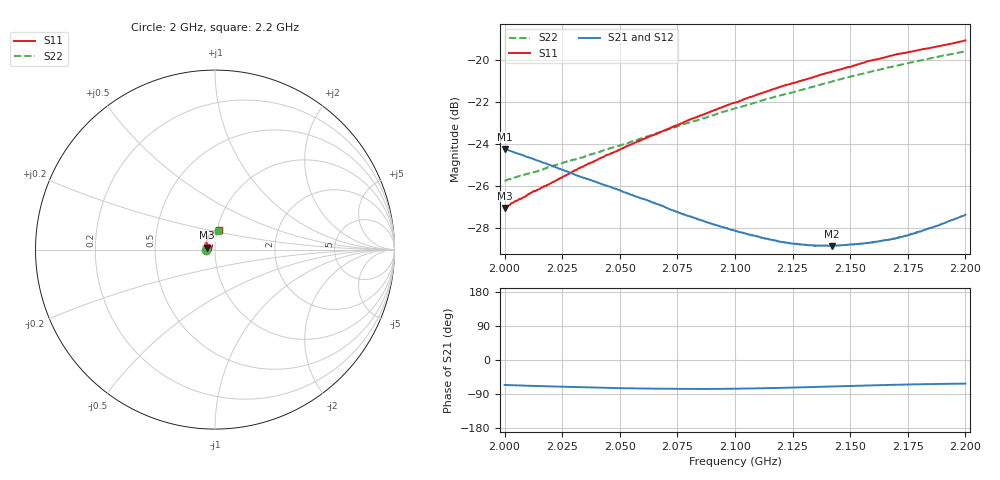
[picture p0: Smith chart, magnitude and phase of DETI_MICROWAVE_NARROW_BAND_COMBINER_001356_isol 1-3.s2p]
! 12/28/2020 4:17:23 PM
! \\DETI-AD\SERVEUR COMMUN\0\01 - PRODUIT\0 01 356 - COMBINEUR 4 VOIES BANDE S 800 WATTS\81 -PROCES VERBAL DE CONTROLE\MESURES\07 - S2P\ISOL 1-3.S2P
! CHANNEL.1
! TR.MEASUREMENT
! CORRECTED.DATA
# GHZ S RI R 50.0
! FREQ.GHZ  S11RE  S11IM  S21RE  S21IM  S12RE  S12IM  S22RE  S22IM
!; PortSelection: Port_12
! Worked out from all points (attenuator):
!   1000 points, 2 GHz to 2.2 GHz, reference 50 ohm
!   highest |S21| = -24.23 dB at 2 GHz (marker M1); lowest = -28.8 dB at 2.142 GHz (marker M2)
!   lowest |S11| = -27.0 dB at 2 GHz (marker M3), VSWR 1.09, Z = 45.9 + j1.04 ohm
!   |S11| at or under -10 dB: start of sweep to end of sweep
!   |S22| runs from -25.7 to -19.6 dB; largest |S21 - S12| = 0.00038
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2  -0.043 0.0113  0.0252 -0.056  0.0252 -0.0562  -0.0517 0.000494
2.011812  -0.0451 0.0178  0.0216 -0.0542  0.0218 -0.0543  -0.0535 0.00736
2.018619  -0.0456 0.0217  0.0199 -0.0529  0.0199 -0.0531  -0.0542 0.0117
2.033433  -0.0467 0.0302  0.0163 -0.0501  0.0163 -0.0504  -0.0548 0.0205
2.044244  -0.0468 0.0366  0.0143 -0.0482  0.0143 -0.0483  -0.0547 0.0275
2.052853  -0.0463 0.0416  0.0129 -0.0466  0.0129 -0.0467  -0.0541 0.0329
2.066667  -0.0448 0.0499  0.0113 -0.044  0.0113 -0.044  -0.0525 0.0418
2.074675  -0.0434 0.0547  0.0105 -0.0423  0.0105 -0.0424  -0.0511 0.0469
2.079279  -0.0426 0.0576  0.0101 -0.0415  0.0102 -0.0417  -0.0501 0.0499
2.1001  -0.037 0.0698  0.0097 -0.0381  0.00975 -0.0383  -0.0441 0.0627
2.116116  -0.0313 0.079  0.0103 -0.0359  0.0102 -0.0361  -0.0376 0.072
2.120521  -0.0295 0.0813  0.0105 -0.0354  0.0104 -0.0356  -0.0357 0.0743
2.128929  -0.0256 0.0853  0.0111 -0.0347  0.0111 -0.0349  -0.0313 0.0787
2.133534  -0.0232 0.0876  0.0115 -0.0344  0.0114 -0.0347  -0.0289 0.0811
2.142142  -0.0188 0.0917  0.0124 -0.034  0.0122 -0.0342  -0.0239 0.0854
2.153353  -0.0119 0.0967  0.0137 -0.0339  0.0138 -0.0339  -0.017 0.0904
2.158358  -0.0088 0.0989  0.0144 -0.0339  0.0143 -0.0341  -0.0137 0.0925
2.166767  -0.00362 0.1018  0.0153 -0.0341  0.0153 -0.0342  -0.00779 0.0955
2.172372  0.000163 0.1034  0.016 -0.0345  0.0162 -0.0344  -0.00379 0.0973
2.181181  0.00647 0.1055  0.0173 -0.0353  0.0172 -0.0354  0.00285 0.0996
2.195596  0.018 0.108  0.0193 -0.0373  0.0193 -0.0374  0.0146 0.1025
2.2  0.0217 0.1088  0.02 -0.038  0.02 -0.0382  0.0183 0.1029
